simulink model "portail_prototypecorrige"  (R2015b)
settings: Solver=FixedStepDiscrete  StartTime=0.0  StopTime=inf  RelTol=1e-3
libraries: arduinolib x6

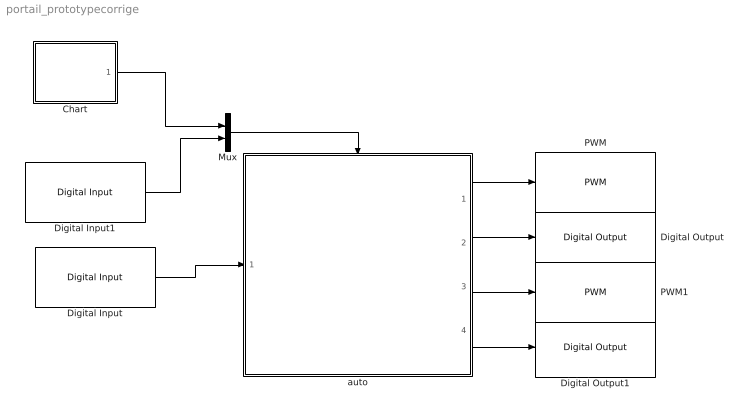
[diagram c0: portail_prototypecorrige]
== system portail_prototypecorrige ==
  Chart : Stateflow chart  TreatAsAtomicUnit=on
  Digital Input : arduinolib/Digital Input  pinNumber=5  sampleTime=0.1  blockPlatform=arduino
  Digital Input1 : arduinolib/Digital Input  pinNumber=6  sampleTime=0.1  blockPlatform=arduino
  Digital Output : arduinolib/Digital Output  pinNumber=12  blockPlatform=arduino
  Digital Output1 : arduinolib/Digital Output  pinNumber=13  blockPlatform=arduino
  Mux : Mux  Inputs=2
  PWM : arduinolib/PWM  pinNumber=3  blockPlatform=arduino
  PWM1 : arduinolib/PWM  pinNumber=11  blockPlatform=arduino
  auto : Stateflow chart  TreatAsAtomicUnit=on
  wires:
  auto/1(CGV) -> PWM/1
  auto/2(SGV) -> Digital Output/1
  auto/4(SPV) -> Digital Output1/1
  auto/3(CPV) -> PWM1/1
  Mux/1 -> auto/Trigger
  Digital Input/1 -> auto/1(encl)
  Digital Input1/1 -> Mux/2
  Chart/1(horl) -> Mux/1

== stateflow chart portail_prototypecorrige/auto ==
  state portail_arrete
    du:CGV=0;
    SGV=0;
    CPV=0;
    SPV=0;
  state portail_marche_auto
    state ouverture
      du:CGV=150;
      SGV=0;
      CPV=150;
      SPV=0;
    state arret
      du:CGV=0;
      SGV=0;
      CPV=0;
      SPV=0;
    state fermeture
      state fermeture_G_V [parallel]
        state fermGV
          du:CGV=150;
          SGV=1;
        (default) -> fermGV
      state fermeture_P_V [parallel]
        state fermPV
          du:CPV=150;
          SPV=1;
        state attentePV
        (default) -> attentePV
        attentePV -> fermPV : after(2,sec)
    state arretbis
      du:CGV=0;
      SGV=0;
      CPV=0;
      SPV=0;
    (default) -> arret
    arret -> ouverture : dem
    fermeture -> arret : after(5,sec)
    ouverture -> arretbis : after(5,sec)
    arretbis -> fermeture : after(4,sec)
  (default) -> portail_arrete
  portail_marche_auto -> portail_arrete : [!encl]
  portail_arrete -> portail_marche_auto : [encl]
  data: CGV output; SGV output; CPV output; SPV output; encl input
  events: input RISING_EDGE_EVENT; input RISING_EDGE_EVENT

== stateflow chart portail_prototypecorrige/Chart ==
  state zero
    entry:horl;
  state un
    entry:horl;
  zero -> un : after(0.1,sec)
  (default) -> zero
  un -> zero : after(0.1,sec)
  events: output EITHER_EDGE_EVENT
